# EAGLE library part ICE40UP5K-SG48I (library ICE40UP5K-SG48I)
FPGA - Field Programmable Gate Array iCE40-UltraPlus, 5280 LUTs, 1.2V Source: Datasheet
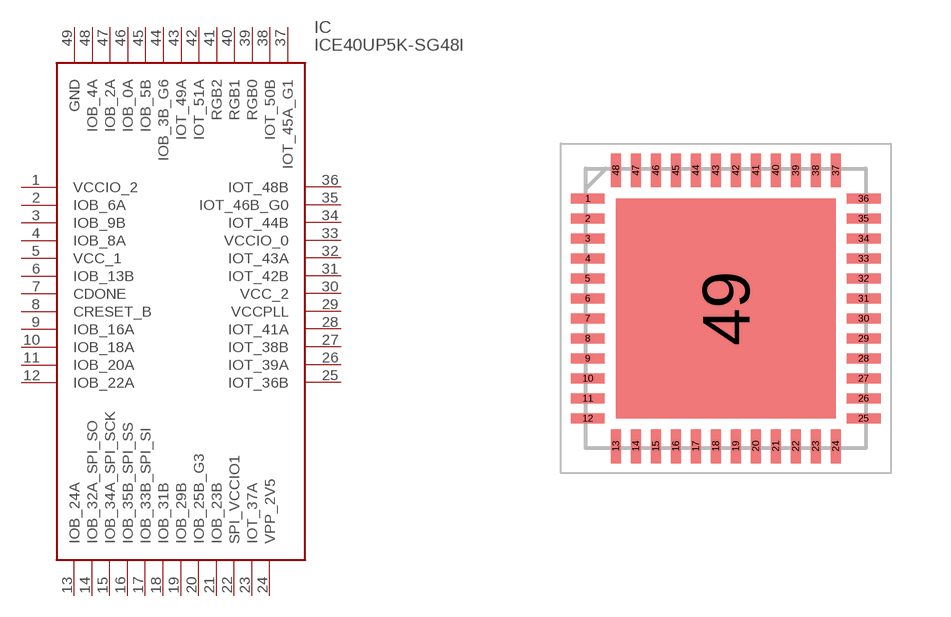
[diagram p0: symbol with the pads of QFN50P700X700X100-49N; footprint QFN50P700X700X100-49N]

Designator prefix IC

## ICE40UP5K-SG48I (Description: FPGA - Field Programmable Gate Array iCE40-UltraPlus, 5280 LUTs, 1.2V; Height: 1mm; Manufacturer_Name: Lattice Semiconductor; Manufacturer_Part_Number: ICE40UP5K-SG48I; Mouser_Part_Number: 842-ICE40UP5K-SG48I; Mouser_Price-Stock: https://www.mouser.co.uk/ProductDetail/Lattice/ICE40UP5K-SG48I?qs=Rp3RbKSfAt3UqOG1AN4%2FAg%3D%3D)  [QFN50P700X700X100-49N]
1  VCCIO_2
2  IOB_6A
3  IOB_9B
4  IOB_8A
5  VCC_1
6  IOB_13B
7  CDONE
8  CRESET_B
9  IOB_16A
10  IOB_18A
11  IOB_20A
12  IOB_22A
13  IOB_24A
14  IOB_32A_SPI_SO
15  IOB_34A_SPI_SCK
16  IOB_35B_SPI_SS
17  IOB_33B_SPI_SI
18  IOB_31B
19  IOB_29B
20  IOB_25B_G3
21  IOB_23B
22  SPI_VCCIO1
23  IOT_37A
24  VPP_2V5
25  IOT_36B
26  IOT_39A
27  IOT_38B
28  IOT_41A
29  VCCPLL
30  VCC_2
31  IOT_42B
32  IOT_43A
33  VCCIO_0
34  IOT_44B
35  IOT_46B_G0
36  IOT_48B
37  IOT_45A_G1
38  IOT_50B
39  RGB0
40  RGB1
41  RGB2
42  IOT_51A
43  IOT_49A
44  IOB_3B_G6
45  IOB_5B
46  IOB_0A
47  IOB_2A
48  IOB_4A
49  GND

## Footprint QFN50P700X700X100-49N (pad centres in mm)
48-Pin QFN
smd 0.85 x 0.25: 1 -3.45,2.75; 2 -3.45,2.25; 3 -3.45,1.75; 4 -3.45,1.25; 5 -3.45,0.75; 6 -3.45,0.25; 7 -3.45,-0.25; 8 -3.45,-0.75; 9 -3.45,-1.25; 10 -3.45,-1.75; 11 -3.45,-2.25; 12 -3.45,-2.75; 25 3.45,-2.75; 26 3.45,-2.25; 27 3.45,-1.75; 28 3.45,-1.25; 29 3.45,-0.75; 30 3.45,-0.25; 31 3.45,0.25; 32 3.45,0.75; 33 3.45,1.25; 34 3.45,1.75; 35 3.45,2.25; 36 3.45,2.75
smd 0.25 x 0.85: 13 -2.75,-3.45; 14 -2.25,-3.45; 15 -1.75,-3.45; 16 -1.25,-3.45; 17 -0.75,-3.45; 18 -0.25,-3.45; 19 0.25,-3.45; 20 0.75,-3.45; 21 1.25,-3.45; 22 1.75,-3.45; 23 2.25,-3.45; 24 2.75,-3.45; 37 2.75,3.45; 38 2.25,3.45; 39 1.75,3.45; 40 1.25,3.45; 41 0.75,3.45; 42 0.25,3.45; 43 -0.25,3.45; 44 -0.75,3.45; 45 -1.25,3.45; 46 -1.75,3.45; 47 -2.25,3.45; 48 -2.75,3.45
smd 5.5 x 5.5: 49 0,0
